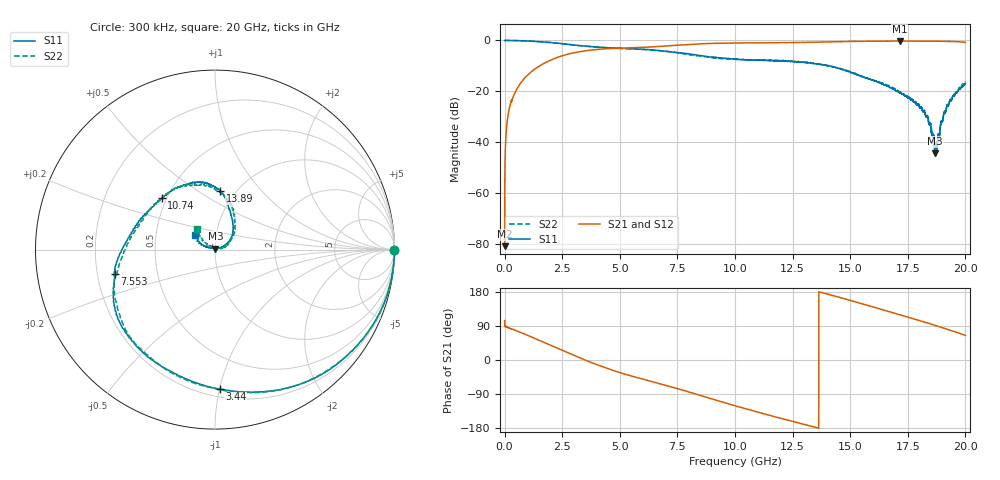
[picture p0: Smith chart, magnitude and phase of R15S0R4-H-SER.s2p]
!{R15S0R4}
!Johanson Technology Inc.
!www.johansontechnology.com
!Test Board Conditions:
!Substrate Type  RO4350B
!Substrate Thickness  20 mil
!Substrate Dk  3.66
!TL Type: GCPW
!TL Trace Width  34 mil
!TL Gap  10 mil
!Electrode orientation  Horizontal
!DUT TOPOLOGY	SERIES
!Mounting Pad LxW  26x52 mil
! Created Sat Feb  6 12:05:34 2021
# hz S ma R 50
! 2 Port Network Data from SP1.SP block
! freq  magS11  angS11  magS21  angS21  magS12  angS12  magS22  angS22
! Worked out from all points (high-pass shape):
!   20001 points, 300 kHz to 20 GHz, reference 50 ohm
!   highest |S21| = -0.19 dB at 17.16 GHz (marker M1); lowest = -80.7 dB at 300 kHz (marker M2)
!   |S21| within 3 dB of the highest: 4.617 GHz to end of sweep
!   lowest |S11| = -44.3 dB at 18.68 GHz (marker M3), VSWR 1.01, Z = 50.2 + j0.582 ohm
!   |S11| at or under -10 dB: 14.08673 GHz to 14.08924 GHz (2.513 MHz wide, 0.0178 % of centre); 14.08939 GHz to 14.09287 GHz (3.482 MHz wide, 0.0247 % of centre); 14.09 GHz to end of sweep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
!   |S22| runs from -45.2 to 0.0 dB; largest |S21 - S12| = 0.013
!   S11 on the Smith chart (normalised r, x): 300 kHz: open; 3.44 GHz: 0.25, -1.00; 7.553 GHz: 0.27, -0.11; 10.74 GHz: 0.47, +0.32; 13.89 GHz: 0.85, +0.62; 20 GHz: 0.79, +0.13
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300000  0.9952 0.0  9.184e-05 103.9  3.878e-05 89.6  0.9957 -0.1
1.013e8  0.9997 -2.7  0.02296 87.1  0.02315 87.1  0.9993 -2.7
1.383e8  0.9993 -3.6  0.03142 86.2  0.03162 86.2  0.9994 -3.6
2.673e8  0.9977 -7.2  0.06078 82.2  0.06101 82.2  0.9973 -7.2
5.203e8  0.9938 -12.7  0.1087 77.0  0.1089 77.2  0.9933 -12.7
1.5523e9  0.9428 -39.3  0.3237 50.6  0.3249 50.6  0.9423 -39.2
3.3343e9  0.786 -85.6  0.6091 3.9  0.6106 3.9  0.7862 -86.2
3.4403e9  0.7776 -88.1  0.6204 1.3  0.6205 1.3  0.778 -89.0
4.9233e9  0.7062 -120.7  0.7019 -31.6  0.7044 -31.6  0.6985 -122.2
6.6673e9  0.6362 -152.4  0.7608 -61.6  0.7634 -61.4  0.6284 -150.3
7.5533e9  0.5754 -166.5  0.8083 -76.3  0.8109 -76.4  0.5673 -165.5
1.00003e10  0.4327 150.5  0.8926 -120.7  0.8945 -120.8  0.4278 149.1
1.07433e10  0.4126 136.1  0.8991 -133.3  0.8975 -133.7  0.4178 137.5
1.33343e10  0.356 91.7  0.9226 -175.2  0.9188 -175.3  0.3579 98.5
1.38873e10  0.3284 85.0  0.9336 175.9  0.9266 176.0  0.333 87.9
1.66673e10  0.1247 39.2  0.9742 127.9  0.9696 128.3  0.1307 37.3
1.71593e10  0.09583 30.9  0.9788 119.1  0.9702 119.6  0.09778 28.7
1.81663e10  0.04014 18.3  0.9703 101.0  0.9678 101.2  0.04037 11.7
1.86843e10  0.006079 72.7  0.968 91.5  0.9645 91.8  0.008408 73.6
1.87883e10  0.009794 135.0  0.9657 89.4  0.9632 89.7  0.01224 115.4
1.92633e10  0.05294 161.5  0.9594 80.0  0.9619 80.4  0.05374 148.9
2e10  0.1389 143.5  0.919 64.9  0.915 64.8  0.1554 131.4
